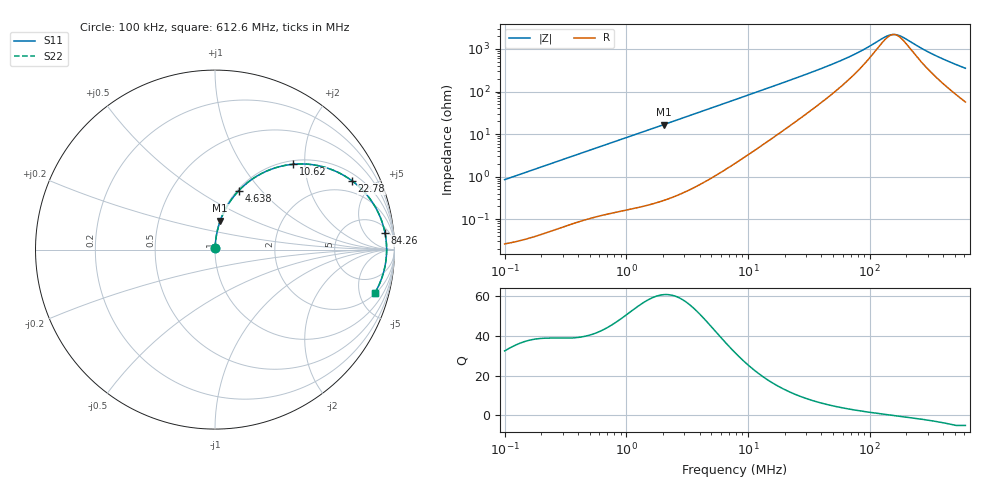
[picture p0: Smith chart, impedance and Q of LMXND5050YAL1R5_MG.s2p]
! LMXND5050YAL1R5_MG  S-PARAMETER MODEL  ( General Type )
! Model Generated by TAIYO YUDEN Corporation (http://www.ty-top.com)
! Version 1.0
! TAIYO YUDEN Control No. 191023NI43SB-FBB
! Copyright(c) 2019 TAIYO YUDEN CO.,LTD. All Rights Reserved.
! Product Description (link to TY-COMPAS)
! https://ds.yuden.co.jp/TYCOMPAS/or/detail?pn=LMXND5050YAL1R5NMG&u=M
! Products Name : Inductors
! Characteristics :
!  Inductance : 1.5 uH , SRF(min) : 60 MHz , DC Resistance(max) : 0.0221 Ohm
!  Rated Current : Saturation :6400 mA , Temp Rise : 4500 mA
!  Case Size : 4.9 x 4.9 / 0.193 x 0.193 [mm/inch] , Thickness : 4.1 / 0.161 [mm/inch]
!  (Conditions: Temperature = 25 degC , DC Bias Current/Voltage = 0A / 0V)
! External Node Assignments :
!  1  o---GGG---o  2
! GND o---------o GND
! Frequency Range : 0.1MHz  -  612.621916MHz  [ 402 STEP ]
# MHz S RI R 50
! Freq[MHz].  S11 Real  S11 Imag  S21 Real  S21 Imag  S12 Real  S12 Imag  S22 Real  S22 Imag
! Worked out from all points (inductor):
!   401 points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, 100 kHz to 612.6 MHz, reference 50 ohm
!   read as one part in series: L = 1.35 uH near 104.5 kHz
!   highest Q = 60.5 at 2.026 MHz (marker M1), where L = 1.31 uH
!   self-resonance near 157.8 MHz
!   S11 on the Smith chart (normalised r, x): 100 kHz: 1.00, +0.02; 4.638 MHz: 1.02, +0.76; 10.62 MHz: 1.07, +1.75; 22.78 MHz: 1.33, +3.78; 84.26 MHz: 8, +16; 612.6 MHz: 2.13, -6.95
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0.1  0.000335 0.00848  0.9997 -0.00848  0.9997 -0.00848  0.000335 0.00848
0.430878  0.0022 0.0359  0.9978 -0.0359  0.9978 -0.0359  0.0022 0.0359
0.965317  0.00787 0.0789  0.9921 -0.0789  0.9921 -0.0789  0.00787 0.0789
1.856562  0.0251 0.1482  0.9749 -0.1482  0.9749 -0.1482  0.0251 0.1482
2.025729  0.0294 0.1609  0.9706 -0.1609  0.9706 -0.1609  0.0294 0.1609
3.201909  0.0683 0.2435  0.9317 -0.2435  0.9317 -0.2435  0.0683 0.2435
4.638363  0.1317 0.3276  0.8683 -0.3276  0.8683 -0.3276  0.1317 0.3276
6.025325  0.2025 0.3892  0.7975 -0.3892  0.7975 -0.3892  0.2025 0.3892
7.827017  0.2982 0.4418  0.7018 -0.4418  0.7018 -0.4418  0.2982 0.4418
10.62057  0.4355 0.4754  0.5645 -0.4754  0.5645 -0.4754  0.4355 0.4754
15.05344  0.6013 0.4614  0.3987 -0.4614  0.3987 -0.4614  0.6013 0.4614
22.77862  0.7639 0.383  0.2361 -0.383  0.2361 -0.383  0.7639 0.383
33.72493  0.8622 0.2847  0.1378 -0.2847  0.1378 -0.2847  0.8622 0.2847
55.68197  0.9251 0.1697  0.0749 -0.1697  0.0749 -0.1697  0.9251 0.1697
84.25705  0.947 0.0938  0.053 -0.0938  0.053 -0.0938  0.947 0.0938
130.3064  0.9555 0.0272  0.0445 -0.0272  0.0445 -0.0272  0.9555 0.0272
145.3134  0.9562 0.0117  0.0438 -0.0117  0.0438 -0.0117  0.9562 0.0117
162.0487  0.9563 -0.00376  0.0437 0.00376  0.0437 0.00376  0.9563 -0.00376
180.7114  0.9559 -0.0192  0.0441 0.0192  0.0441 0.0192  0.9559 -0.0192
332.7278  0.9426 -0.1139  0.0574 0.1139  0.0574 0.1139  0.9426 -0.1139
461.4331  0.9227 -0.1762  0.0773 0.1762  0.0773 0.1762  0.9227 -0.1762
612.6219  0.8922 -0.2392  0.1078 0.2392  0.1078 0.2392  0.8922 -0.2392
